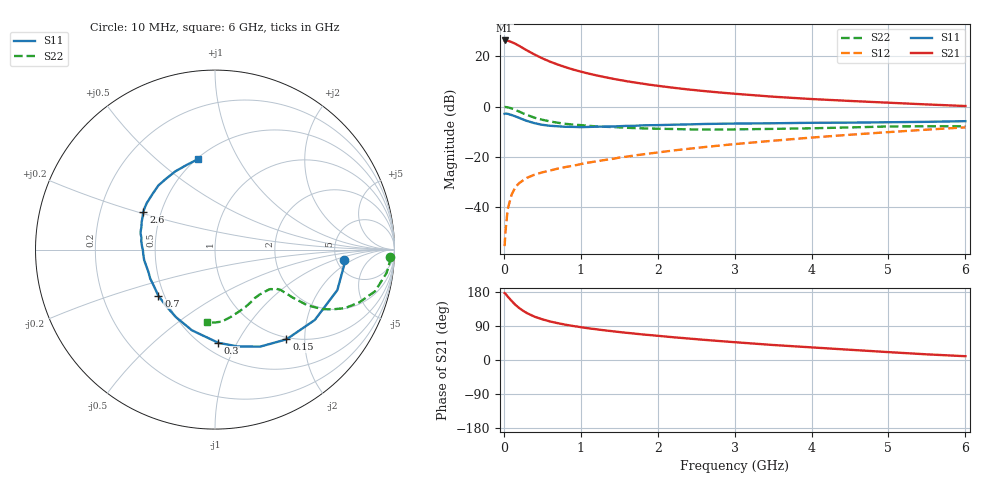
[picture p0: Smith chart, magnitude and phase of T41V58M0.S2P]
! Infineon Technologies  Discrete & RF Semiconductors
! BFR182T
! Si NPN RF Bipolar Junction Transistor in SC75
! VCE = 1.5 V  IC = 8 mA
! Common Emitter S-Parameters:  October  1999
# GHz  S  MA  R  50
!  f  S11  S21  S12  S22
! GHz  MAG  ANG  MAG  ANG  MAG  ANG  MAG  ANG
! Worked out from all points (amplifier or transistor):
!   36 points, 10 MHz to 6 GHz, reference 50 ohm
!   highest |S21| = 26.2 dB at 10 MHz (marker M1)
!   |S21| within 3 dB of that: start of sweep to 247.1 MHz
!   unconditionally stable (mu >= 1): 1.035 GHz to 3.939 GHz
!   at 250 MHz: K = 0.41, MSG = 26.2 dB, |S12| = -29.3 dB
!   at 1.4 GHz: K = 1.09, MAG = 14.2 dB, |S12| = -20.8 dB
!   at 6 GHz: K = 0.85, MSG = 4.2 dB, |S12| = -8.3 dB
!   lowest NFmin = 1.40 dB at 450 MHz
!   S11 on the Smith chart (normalised r, x): 10 MHz: 5.76, -1.44; 150 MHz: 0.97, -1.63; 300 MHz: 0.59, -0.84; 700 MHz: 0.46, -0.29; 2.6 GHz: 0.40, +0.21; 6 GHz: 0.51, +0.70
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0.01  0.7193 -4.8  20.5 176.7  0.0017 84.2  0.9751 -2.4
0.02  0.7264 -6.0  20.45 175.2  0.0031 87.1  0.9803 -3.0
0.05  0.718 -18.3  20.24 167.5  0.0092 86.4  0.9652 -7.7
0.1  0.6803 -35.2  19.07 156.2  0.0177 75.3  0.9216 -14.6
0.15  0.6391 -51.5  17.59 145.6  0.0252 67.2  0.8557 -20.1
0.2  0.5961 -65.1  15.99 137.1  0.0304 64.6  0.7949 -24.2
0.25  0.5541 -76.8  14.42 129.9  0.0343 60.0  0.7337 -27.0
0.3  0.5195 -88.0  13.01 123.8  0.0386 57.7  0.684 -29.0
0.4  0.4678 -105.9  10.77 114.2  0.0445 55.6  0.6012 -31.1
0.5  0.4348 -120.0  9.07 107.4  0.0496 55.0  0.5475 -31.4
0.6  0.4157 -131.4  7.783 101.7  0.0538 55.4  0.5078 -31.7
0.7  0.4069 -140.9  6.82 97.2  0.0588 56.1  0.4774 -31.6
0.9  0.3954 -156.0  5.431 89.8  0.0669 58.0  0.4382 -31.6
1.1  0.3943 -167.5  4.521 83.6  0.0775 59.6  0.4156 -32.2
1.3  0.4006 -176.4  3.873 78.5  0.0867 61.2  0.398 -33.3
1.6  0.4139 173.3  3.18 71.7  0.1018 62.8  0.3795 -35.4
2.2  0.4367 159.3  2.366 60.1  0.1344 64.0  0.359 -42.4
2.6  0.4514 152.2  2.034 53.3  0.1567 64.1  0.3511 -47.8
3.5  0.4663 138.1  1.57 39.6  0.2102 62.2  0.3609 -61.2
4.5  0.4798 124.7  1.293 27.0  0.2762 58.0  0.3856 -77.0
5.5  0.4979 108.2  1.102 14.9  0.3486 52.3  0.4066 -90.7
6  0.5133 100.4  1.025 10.0  0.3867 48.5  0.4053 -96.5
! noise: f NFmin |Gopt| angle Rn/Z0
0.45  1.4  0.26  41  0.29
0.9  1.5  0.25  83  0.23
1.8  2  0.21  162  0.2
